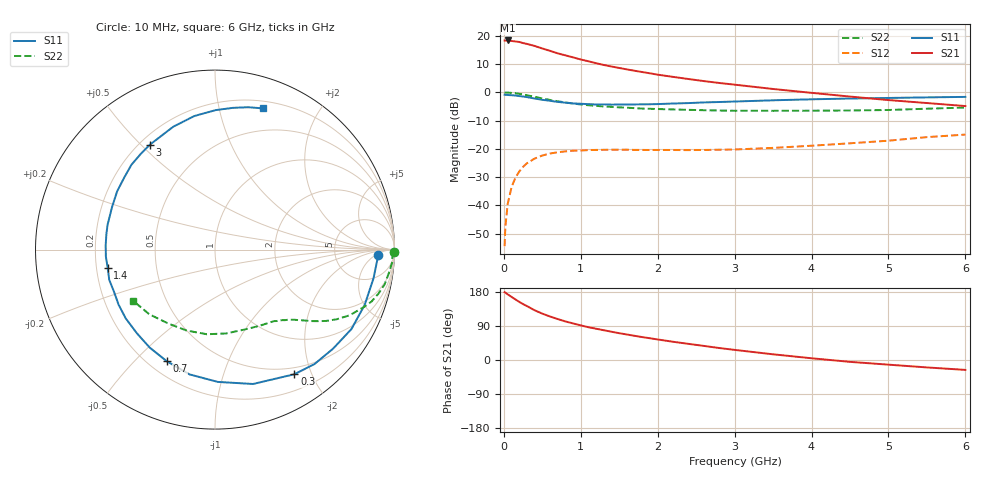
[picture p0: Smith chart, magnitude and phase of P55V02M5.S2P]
! SIEMENS Small Signal Semiconductors
! BFP183
! Si NPN RF Bipolar Junction Transistor in SOT143
! VCE = 5 V  IC = 2.5 mA
! Common Emitter S-Parameters:  March  1996
# GHz  S  MA  R  50
!  f  S11  S21  S12  S22
! GHz  MAG  ANG  MAG  ANG  MAG  ANG  MAG  ANG
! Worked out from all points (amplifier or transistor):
!   36 points, 10 MHz to 6 GHz, reference 50 ohm
!   highest |S21| = 18.4 dB at 50 MHz (marker M1)
!   |S21| within 3 dB of that: start of sweep to 519.8 MHz
!   unconditionally stable (mu >= 1): 1.992 GHz to 5.847 GHz
!   at 250 MHz: K = 0.13, MSG = 21.9 dB, |S12| = -26.4 dB
!   at 1.4 GHz: K = 0.72, MSG = 14.7 dB, |S12| = -20.3 dB
!   at 6 GHz: K = 0.98, MSG = 5.0 dB, |S12| = -14.9 dB
!   S11 on the Smith chart (normalised r, x): 10 MHz: 19, -6; 300 MHz: 0.41, -1.75; 700 MHz: 0.27, -0.62; 1.4 GHz: 0.25, -0.08; 3 GHz: 0.24, +0.53; 6 GHz: 0.27, +1.36
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0.01  0.9087 -1.9  8.277 178.8  0.0019 88.8  0.9968 -0.8
0.02  0.9051 -4.0  8.234 177.8  0.0042 89.9  0.9881 -1.6
0.05  0.8977 -10.2  8.28 173.2  0.0106 87.9  0.9903 -3.9
0.1  0.889 -20.3  8.107 166.6  0.021 78.7  0.9771 -7.8
0.2  0.8587 -40.0  7.797 153.4  0.0397 67.9  0.943 -15.1
0.25  0.8449 -49.0  7.444 147.5  0.0481 63.6  0.9186 -18.4
0.3  0.8234 -57.5  7.192 142.3  0.0556 58.9  0.889 -21.1
0.4  0.7781 -74.2  6.62 131.3  0.0674 50.9  0.8348 -26.0
0.5  0.7373 -88.8  5.975 122.3  0.0763 44.0  0.7798 -29.9
0.6  0.7096 -101.6  5.425 114.8  0.0827 38.7  0.7341 -32.8
0.7  0.6777 -113.3  4.9 108.1  0.0871 34.4  0.695 -35.0
0.8  0.6561 -123.6  4.512 101.8  0.0903 30.5  0.6632 -36.9
0.9  0.6378 -133.0  4.159 96.5  0.0927 27.9  0.6339 -38.5
1.1  0.6187 -150.2  3.545 86.5  0.0952 23.1  0.5911 -41.4
1.4  0.6065 -170.4  2.865 74.6  0.0965 18.2  0.5531 -45.3
1.8  0.6144 166.9  2.286 60.4  0.0958 16.0  0.5163 -50.5
2.2  0.6345 149.3  1.878 48.1  0.0954 15.3  0.4986 -56.6
3  0.688 121.8  1.368 26.7  0.0976 18.9  0.4728 -71.7
3.5  0.7234 108.7  1.147 15.0  0.1041 21.9  0.4712 -82.5
4.5  0.7772 89.7  0.842 -4.9  0.1255 24.8  0.4779 -109.3
5.5  0.8145 76.9  0.647 -19.6  0.1614 23.8  0.5137 -135.5
6  0.8311 71.2  0.572 -26.1  0.179 20.5  0.5381 -148.0
